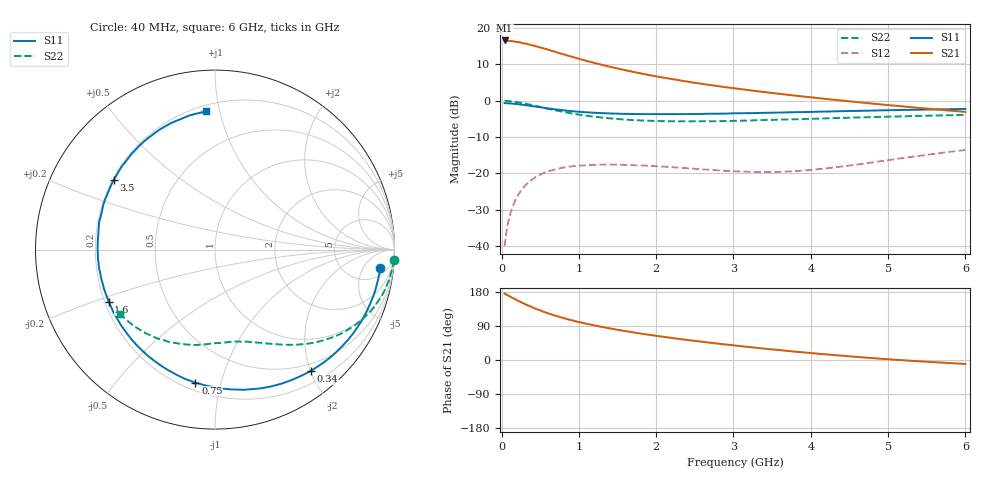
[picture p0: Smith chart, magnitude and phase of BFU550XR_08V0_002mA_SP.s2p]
! Filename:  P:\Prog\Test\Noise\ATS_data\Testdata_Net\03 Spar\BFU550XR_APG2013_45_C05_08p0V_002mA_SP_CM01_D.s2p
! Date/Time: Tue 06/Aug/2013 14:38:17
! BFU550XR_APG2013_45_C05_08p0V_1to35mA_SP_CM01_Bias2_R.s2p
! MDIF S-parameter v. bias file
! BFU550XR_APG2013_45_C05_08p0V_1to35mA_SP_CM01
! Date/time Fri Aug 02 14:53:20 2013
! VAR V_out= 8.0010
! VAR I_out= 2.0050
! VAR V_in= 0.7899
! VAR I_in= 0.0209
! Device data file deembeded for feedlines and parallel
! Original file: \03 Spar\BFU550XR_APG2013_45_C05_08p0V_002mA_SP_CM01_R.s2p
! Feed-files: PR006V01_02082013_Feed1.s2p, PR006V01_02082013_Feed2.s2p
! Parallel-file: PR006V01_02082013_Par.s2p
# MHz S MA R 50
!  Freq-MHz  S11-mag  S11-arg  S21-mag  S21-arg  S12-mag  S12-arg  S22-mag  S22-arg
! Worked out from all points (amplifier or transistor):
!   98 points, 40 MHz to 6 GHz, reference 50 ohm
!   highest |S21| = 16.6 dB at 40 MHz (marker M1)
!   |S21| within 3 dB of that: start of sweep to 671 MHz
!   unconditionally stable (mu >= 1): 3.07 GHz to 4.568 GHz
!   at 300 MHz: K = 0.10, MSG = 19.7 dB, |S12| = -23.5 dB
!   at 1.6 GHz: K = 0.49, MSG = 13.1 dB, |S12| = -17.7 dB
!   at 6 GHz: K = 0.78, MSG = 5.3 dB, |S12| = -13.6 dB
!   S11 on the Smith chart (normalised r, x): 40 MHz: 8, -12; 340 MHz: 0.38, -2.01; 750 MHz: 0.25, -0.83; 1.6 GHz: 0.22, -0.22; 3.5 GHz: 0.20, +0.30; 6 GHz: 0.24, +0.91
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40  0.9263 -6.4  6.78 175.5  0.00989 86.0  0.9964 -3.2
50  0.9255 -7.9  6.779 173.7  0.01229 85.0  0.9953 -4.2
100  0.9198 -15.9  6.671 168.6  0.02437 80.3  0.9868 -8.5
120  0.9161 -19.1  6.688 166.3  0.02906 78.4  0.9836 -10.2
220  0.8952 -34.4  6.439 155.8  0.05112 69.5  0.9502 -18.2
320  0.8664 -48.9  6.125 146.0  0.07009 61.3  0.9074 -25.4
340  0.8614 -51.6  6.044 144.2  0.07339 59.8  0.8978 -26.7
440  0.8306 -64.7  5.665 135.5  0.08844 52.8  0.8511 -32.8
550  0.7982 -78.0  5.254 126.9  0.1011 46.0  0.7986 -38.7
600  0.7837 -83.6  5.079 123.3  0.1058 43.3  0.7768 -41.0
750  0.7494 -98.4  4.519 113.7  0.117 36.3  0.7196 -47.1
900  0.7201 -111.5  4.071 105.2  0.1244 30.4  0.6722 -52.1
1050  0.6996 -122.7  3.665 97.8  0.1282 25.6  0.6311 -56.6
1300  0.6747 -138.4  3.128 87.2  0.1315 19.4  0.5858 -62.8
1600  0.66 -153.8  2.64 76.3  0.1305 14.1  0.5504 -69.3
2050  0.6538 -172.2  2.122 62.5  0.124 9.8  0.524 -77.8
2500  0.6552 172.7  1.768 50.4  0.1154 8.8  0.5207 -85.9
3100  0.6731 155.5  1.444 36.5  0.1058 14.1  0.5309 -96.4
3500  0.6844 145.4  1.28 28.0  0.1044 20.4  0.5453 -103.5
4100  0.7069 131.5  1.087 16.5  0.1141 30.6  0.5671 -113.8
5200  0.747 108.6  0.8343 -0.8  0.1629 38.9  0.6104 -132.5
6000  0.7713 93.9  0.7033 -10.3  0.2093 36.3  0.6389 -145.8
